FUNCTION "Cells_Status" : VOID
TITLE =
VERSION : 0.1


VAR_INPUT
  Start : BOOL ;
  Testing_1 : BOOL ;
  Testing_2 : BOOL ;
  Testing_3 : BOOL ;
  Testing_4 : BOOL ;
  Testing_5 : BOOL ;
  Testing_6 : BOOL ;
END_VAR
VAR_OUTPUT
  Cell_1_result : BOOL ;
  Cell_2_result : BOOL ;
  Cell_3_result : BOOL ;
  Cell_4_result : BOOL ;
  Cell_5_result : BOOL ;
  Cell_6_result : BOOL ;
END_VAR
BEGIN
NETWORK
TITLE =

END_FUNCTION

